| / 7\'7
| \ \   Xilinx Inc.
| / /
| \_\/.\   IBIS Models for VIRTEX-5
[IBIS ver]   3.2
[File name]   dlpc950.ibs
[File Rev]   2.6
[Date]   Tue August 11 14:17:33 2015
[Source]   Derived from spice models, rev0.20, dated 08/17/2007 using
   hspice 2005.03
[Notes]   Xilinx IBIS file for VIRTEX-5 I/O standards.
   All models are preliminary.
   The version of IBISCHK used is ibischk4.
   Ibis models were generated using S2IBIS3.
[Disclaimer] The data in this file is derived from SPICE simulations using
   modeling information extracted from the target process. While
   a great deal of care has been taken to provide information
   that is accurate, this model is considered preliminary as it
   has not been verified by actual silicon measurement. Treat the
   data in this model as preliminary until actual silicon
   verification is performed.
[Copyright]   Copyright 2007, Xilinx Inc., All rights reserved
|   Component VIRTEX-5
[Component]   VIRTEX-5
[Manufacturer]   Xilinx Inc.
[Package]
|FF676
|variable   typ   min   max
R_pkg   311.14m   20.66m   859.35m
L_pkg   3.55nH   0.59nH   9.38nH
C_pkg   2.19pF   0.88pF   4.60pF
[Pin]  signal_name   model_name   R_pin   L_pin   C_pin
G11   dmd_type<0>   LVCMOS25_S_12
G12   dmd_type<1>   LVCMOS25_S_12
H11   dmd_type<2>   LVCMOS25_S_12
H12   dmd_type<3>   LVCMOS25_S_12
AC7   scpclk   LVDCI_33
G10   rst_active   LVCMOS25_S_12
D25   ddcspare0   LVCMOS25_S_12
D26   ddcspare1   LVCMOS25_S_12
B21   dclkin_an   LVDS_25
A7   dclkin_bn   LVDS_25
C21   dclkin_ap   LVDS_25
K20   dclkin_cn   LVDS_25
B7   dclkin_bp   LVDS_25
L5   dclkin_dn   LVDS_25
K21   dclkin_cp   LVDS_25
K5   dclkin_dp   LVDS_25
AD10   reset_strobe   LVDCI_33
A15   din_an<0>   LVDS_25
B14   din_an<1>   LVDS_25
B16   din_an<2>   LVDS_25
C16   din_an<3>   LVDS_25
A17   din_an<4>   LVDS_25
C17   din_an<5>   LVDS_25
A19   din_an<6>   LVDS_25
C18   din_an<7>   LVDS_25
A12   din_bn<0>   LVDS_25
A14   din_ap<0>   LVDS_25
D19   din_an<8>   LVDS_25
B12   din_bn<1>   LVDS_25
C14   din_ap<1>   LVDS_25
B20   din_an<9>   LVDS_25
D10   din_bn<2>   LVDS_25
B15   din_ap<2>   LVDS_25
C12   din_bn<3>   LVDS_25
D16   din_ap<3>   LVDS_25
A10   din_bn<4>   LVDS_25
B17   din_ap<4>   LVDS_25
D9   din_bn<5>   LVDS_25
D18   din_ap<5>   LVDS_25
B10   din_bn<6>   LVDS_25
A18   din_ap<6>   LVDS_25
A8   din_bn<7>   LVDS_25
B19   din_ap<7>   LVDS_25
E20   din_cn<0>   LVDS_25
A13   din_bp<0>   LVDS_25
D6   din_bn<8>   LVDS_25
C19   din_ap<8>   LVDS_25
F20   din_cn<1>   LVDS_25
C13   din_bp<1>   LVDS_25
C7   din_bn<9>   LVDS_25
A20   din_ap<9>   LVDS_25
H19   din_cn<2>   LVDS_25
D11   din_bp<2>   LVDS_25
E23   din_cn<3>   LVDS_25
C11   din_bp<3>   LVDS_25
F23   din_cn<4>   LVDS_25
B11   din_bp<4>   LVDS_25
G22   din_cn<5>   LVDS_25
C9   din_bp<5>   LVDS_25
J20   din_cn<6>   LVDS_25
B9   din_bp<6>   LVDS_25
H22   din_cn<7>   LVDS_25
A9   din_bp<7>   LVDS_25
T3   din_dn<0>   LVDS_25
E21   din_cp<0>   LVDS_25
J23   din_cn<8>   LVDS_25
D5   din_bp<8>   LVDS_25
R5   din_dn<1>   LVDS_25
G20   din_cp<1>   LVDS_25
K22   din_cn<9>   LVDS_25
C6   din_bp<9>   LVDS_25
R7   din_dn<2>   LVDS_25
J19   din_cp<2>   LVDS_25
N3   din_dn<3>   LVDS_25
E22   din_cp<3>   LVDS_25
P4   din_dn<4>   LVDS_25
F22   din_cp<4>   LVDS_25
N6   din_dn<5>   LVDS_25
G21   din_cp<5>   LVDS_25
N4   din_dn<6>   LVDS_25
J21   din_cp<6>   LVDS_25
M7   din_dn<7>   LVDS_25
H21   din_cp<7>   LVDS_25
R3   din_dp<0>   LVDS_25
K7   din_dn<8>   LVDS_25
H23   din_cp<8>   LVDS_25
R6   din_dp<1>   LVDS_25
J4   din_dn<9>   LVDS_25
K23   din_cp<9>   LVDS_25
P6   din_dp<2>   LVDS_25
P3   din_dp<3>   LVDS_25
P5   din_dp<4>   LVDS_25
N7   din_dp<5>   LVDS_25
M4   din_dp<6>   LVDS_25
L7   din_dp<7>   LVDS_25
K6   din_dp<8>   LVDS_25
J5   din_dp<9>   LVDS_25
AD8   reset_irqz   LVCMOS33_S_12
AA10   iic_addr_sel   LVCMOS33_S_12
N1   dclk_an   LVDS_25
Y5   dclk_bn   LVDS_25
M1   dclk_ap   LVDS_25
AA22   dclk_cn   LVDS_25
Y6   dclk_bp   LVDS_25
M26   dclk_dn   LVDS_25
AB22   dclk_cp   LVDS_25
M25   dclk_dp   LVDS_25
H8   speed_sel<0>   LVCMOS25_S_12
H9   speed_sel<1>   LVCMOS25_S_12
G19   comp_data   LVCMOS25_S_12
AA8   iic_sda   LVCMOS33_S_12
E10   clk_r   LVCMOS25_S_12
Y8   iic_scl   LVCMOS33_S_12
F9   arstz   LVCMOS25_S_12
AC8   scpdi   LVCMOS33_S_12
D20   dvalid_an   LVDS_25
C8   dvalid_bn   LVDS_25
D21   dvalid_ap   LVDS_25
L19   dvalid_cn   LVDS_25
D8   dvalid_bp   LVDS_25
L3   dvalid_dn   LVDS_25
L20   dvalid_cp   LVDS_25
L4   dvalid_dp   LVDS_25
F19   ns_flip   LVCMOS25_S_12
A22   din_an<10>   LVDS_25
A24   din_an<11>   LVDS_25
C23   din_an<12>   LVDS_25
C24   din_an<13>   LVDS_25
A25   din_an<14>   LVDS_25
C26   din_an<15>   LVDS_25
B6   din_bn<10>   LVDS_25
B22   din_ap<10>   LVDS_25
D4   din_bn<11>   LVDS_25
A23   din_ap<11>   LVDS_25
B4   din_bn<12>   LVDS_25
B24   din_ap<12>   LVDS_25
C3   din_bn<13>   LVDS_25
D24   din_ap<13>   LVDS_25
A3   din_bn<14>   LVDS_25
B25   din_ap<14>   LVDS_25
B2   din_bn<15>   LVDS_25
B26   din_ap<15>   LVDS_25
M19   din_cn<10>   LVDS_25
B5   din_bp<10>   LVDS_25
M21   din_cn<11>   LVDS_25
D3   din_bp<11>   LVDS_25
N19   din_cn<12>   LVDS_25
C4   din_bp<12>   LVDS_25
N21   din_cn<13>   LVDS_25
C2   din_bp<13>   LVDS_25
P20   din_cn<14>   LVDS_25
A2   din_bp<14>   LVDS_25
N23   din_cn<15>   LVDS_25
B1   din_bp<15>   LVDS_25
H7   din_dn<10>   LVDS_25
M20   din_cp<10>   LVDS_25
G4   din_dn<11>   LVDS_25
M22   din_cp<11>   LVDS_25
G5   din_dn<12>   LVDS_25
P19   din_cp<12>   LVDS_25
G7   din_dn<13>   LVDS_25
N22   din_cp<13>   LVDS_25
F4   din_dn<14>   LVDS_25
P21   din_cp<14>   LVDS_25
E5   din_dn<15>   LVDS_25
P23   din_cp<15>   LVDS_25
J6   din_dp<10>   LVDS_25
H4   din_dp<11>   LVDS_25
H6   din_dp<12>   LVDS_25
G6   din_dp<13>   LVDS_25
F5   din_dp<14>   LVDS_25
E6   din_dp<15>   LVDS_25
AA9   reserved<0>   LVCMOS33_S_12
Y10   reserved<1>   LVCMOS33_S_12
Y11   reserved<2>   LVCMOS33_S_12
AB11   reserved<3>   LVCMOS33_S_12
F18   version<0>   LVCMOS25_S_12
G17   version<1>   LVCMOS25_S_12
H18   version<2>   LVCMOS25_S_12
E1   tstpt_u<10>   LVCMOS25_S_12
E2   tstpt_u<11>   LVCMOS25_S_12
E3   tstpt_u<12>   LVCMOS25_S_12
F3   tstpt_u<13>   LVCMOS25_S_12
E7   tstpt_u<14>   LVCMOS25_S_12
F7   tstpt_u<15>   LVCMOS25_S_12
AD11   dad_spare_scpenz   LVCMOS33_S_12
AC9   scpdo   LVDCI_33
AA17   led0   LVCMOS33_S_12
AB17   led1   LVCMOS33_S_12
E12   blkad<0>   LVCMOS25_S_12
D13   blkad<1>   LVCMOS25_S_12
E13   blkad<2>   LVCMOS25_S_12
F13   blkad<3>   LVCMOS25_S_12
K1   dout_an<10>   LVDS_25
K2   dout_an<11>   LVDS_25
J3   dout_an<12>   LVDS_25
H2   dout_an<13>   LVDS_25
H1   dout_an<14>   LVDS_25
G2   dout_an<15>   LVDS_25
W6   dout_bn<10>   LVDS_25
L2   dout_ap<10>   LVDS_25
V7   dout_bn<11>   LVDS_25
K3   dout_ap<11>   LVDS_25
U4   dout_bn<12>   LVDS_25
H3   dout_ap<12>   LVDS_25
T4   dout_bn<13>   LVDS_25
J1   dout_ap<13>   LVDS_25
U6   dout_bn<14>   LVDS_25
G1   dout_ap<14>   LVDS_25
U7   dout_bn<15>   LVDS_25
F2   dout_ap<15>   LVDS_25
Y20   dout_cn<10>   LVDS_25
W5   dout_bp<10>   LVDS_25
AA24   dout_cn<11>   LVDS_25
V6   dout_bp<11>   LVDS_25
AA19   dout_cn<12>   LVDS_25
V3   dout_bp<12>   LVDS_25
AC24   dout_cn<13>   LVDS_25
T5   dout_bp<13>   LVDS_25
AC19   dout_cn<14>   LVDS_25
U5   dout_bp<14>   LVDS_25
AC22   dout_cn<15>   LVDS_25
T7   dout_bp<15>   LVDS_25
L25   dout_dn<10>   LVDS_25
Y21   dout_cp<10>   LVDS_25
K26   dout_dn<11>   LVDS_25
AA23   dout_cp<11>   LVDS_25
J26   dout_dn<12>   LVDS_25
AA20   dout_cp<12>   LVDS_25
J24   dout_dn<13>   LVDS_25
AB24   dout_cp<13>   LVDS_25
H26   dout_dn<14>   LVDS_25
AD19   dout_cp<14>   LVDS_25
G25   dout_dn<15>   LVDS_25
AC23   dout_cp<15>   LVDS_25
L24   dout_dp<10>   LVDS_25
K25   dout_dp<11>   LVDS_25
J25   dout_dp<12>   LVDS_25
H24   dout_dp<13>   LVDS_25
G26   dout_dp<14>   LVDS_25
G24   dout_dp<15>   LVDS_25
H13   blkmd<0>   LVCMOS25_S_12
H14   blkmd<1>   LVCMOS25_S_12
AB9   dmdscpenz   LVDCI_33
G16   rowad<10>   LVCMOS25_S_12
AB10   dmd_a_reset   LVDCI_33
E26   init_active   LVCMOS25_S_12
AD18   reset_addr<0>   LVDCI_33
AC18   reset_addr<1>   LVDCI_33
AC17   reset_addr<2>   LVDCI_33
AC16   reset_addr<3>   LVDCI_33
E25   ecp2_finished   LVCMOS25_S_12
E8   vsp_en   LVCMOS25_S_12
Y12   tstpt_u<0>   LVCMOS33_S_12
AA12   tstpt_u<1>   LVCMOS33_S_12
Y13   tstpt_u<2>   LVCMOS33_S_12
AA13   tstpt_u<3>   LVCMOS33_S_12
AA14   tstpt_u<4>   LVCMOS33_S_12
AB14   tstpt_u<5>   LVCMOS33_S_12
AA15   tstpt_u<6>   LVCMOS33_S_12
AB15   tstpt_u<7>   LVCMOS33_S_12
C1   tstpt_u<8>   LVCMOS25_S_12
D1   tstpt_u<9>   LVCMOS25_S_12
G9   pwr_float   LVCMOS25_S_12
AD14   reset_oez   LVDCI_33
AE2   dout_an<0>   LVDS_25
AD1   dout_an<1>   LVDS_25
AC1   dout_an<2>   LVDS_25
AB1   dout_an<3>   LVDS_25
Y2   dout_an<4>   LVDS_25
W1   dout_an<5>   LVDS_25
V1   dout_an<6>   LVDS_25
U1   dout_an<7>   LVDS_25
AC13   reset_mode<0>   LVDCI_33
AE5   dout_bn<0>   LVDS_25
AF2   dout_ap<0>   LVDS_25
R2   dout_an<8>   LVDS_25
AD13   reset_mode<1>   LVDCI_33
F25   wdt_enablez   LVCMOS25_S_12
AD3   dout_bn<1>   LVDS_25
AE1   dout_ap<1>   LVDS_25
N2   dout_an<9>   LVDS_25
AD5   dout_bn<2>   LVDS_25
AC2   dout_ap<2>   LVDS_25
AC3   dout_bn<3>   LVDS_25
AB2   dout_ap<3>   LVDS_25
AB5   dout_bn<4>   LVDS_25
AA2   dout_ap<4>   LVDS_25
AB7   dout_bn<5>   LVDS_25
Y1   dout_ap<5>   LVDS_25
AA5   dout_bn<6>   LVDS_25
V2   dout_ap<6>   LVDS_25
AA7   dout_bn<7>   LVDS_25
U2   dout_ap<7>   LVDS_25
T22   dout_cn<0>   LVDS_25
AE6   dout_bp<0>   LVDS_25
Y3   dout_bn<8>   LVDS_25
T2   dout_ap<8>   LVDS_25
R20   dout_cn<1>   LVDS_25
AD4   dout_bp<1>   LVDS_25
W4   dout_bn<9>   LVDS_25
M2   dout_ap<9>   LVDS_25
T19   dout_cn<2>   LVDS_25
AD6   dout_bp<2>   LVDS_25
U21   dout_cn<3>   LVDS_25
AC4   dout_bp<3>   LVDS_25
U20   dout_cn<4>   LVDS_25
AB6   dout_bp<4>   LVDS_25
V23   dout_cn<5>   LVDS_25
AC6   dout_bp<5>   LVDS_25
V22   dout_cn<6>   LVDS_25
AA4   dout_bp<6>   LVDS_25
W19   dout_cn<7>   LVDS_25
Y7   dout_bp<7>   LVDS_25
AB26   dout_dn<0>   LVDS_25
T23   dout_cp<0>   LVDS_25
W23   dout_cn<8>   LVDS_25
W3   dout_bp<8>   LVDS_25
AA25   dout_dn<1>   LVDS_25
R21   dout_cp<1>   LVDS_25
Y22   dout_cn<9>   LVDS_25
V4   dout_bp<9>   LVDS_25
Y26   dout_dn<2>   LVDS_25
T20   dout_cp<2>   LVDS_25
W26   dout_dn<3>   LVDS_25
U22   dout_cp<3>   LVDS_25
U26   dout_dn<4>   LVDS_25
U19   dout_cp<4>   LVDS_25
U25   dout_dn<5>   LVDS_25
V24   dout_cp<5>   LVDS_25
T25   dout_dn<6>   LVDS_25
V21   dout_cp<6>   LVDS_25
R26   dout_dn<7>   LVDS_25
V19   dout_cp<7>   LVDS_25
AC26   dout_dp<0>   LVDS_25
P24   dout_dn<8>   LVDS_25
W24   dout_cp<8>   LVDS_25
AB25   dout_dp<1>   LVDS_25
N24   dout_dn<9>   LVDS_25
Y23   dout_cp<9>   LVDS_25
Y25   dout_dp<2>   LVDS_25
W25   dout_dp<3>   LVDS_25
V26   dout_dp<4>   LVDS_25
U24   dout_dp<5>   LVDS_25
T24   dout_dp<6>   LVDS_25
R25   dout_dp<7>   LVDS_25
P25   dout_dp<8>   LVDS_25
M24   dout_dp<9>   LVDS_25
E18   rst2blkz   LVCMOS25_S_12
R1   sctrl_an   LVDS_25
AA3   sctrl_bn   LVDS_25
P1   sctrl_ap   LVDS_25
W20   sctrl_cn   LVDS_25
AB4   sctrl_bp   LVDS_25
N26   sctrl_dn   LVDS_25
W21   sctrl_cp   LVDS_25
P26   sctrl_dp   LVDS_25
D14   rowad<0>   LVCMOS25_S_12
D15   rowad<1>   LVCMOS25_S_12
E15   rowad<2>   LVCMOS25_S_12
F14   rowad<3>   LVCMOS25_S_12
G14   rowad<4>   LVCMOS25_S_12
E16   rowad<5>   LVCMOS25_S_12
F15   rowad<6>   LVCMOS25_S_12
G15   rowad<7>   LVCMOS25_S_12
E17   rowad<8>   LVCMOS25_S_12
F17   rowad<9>   LVCMOS25_S_12
H17   rowmd<0>   LVCMOS25_S_12
H16   rowmd<1>   LVCMOS25_S_12
AD15   reset_sel<0>   LVDCI_33
AC14   reset_sel<1>   LVDCI_33
AC12   dad_scpenz   LVCMOS33_S_12
F8   reserved_clk   LVCMOS25_S_12
N14   VP_0   NC
P13   VN_0   NC
AA18   A25   LVCMOS25_F_12
Y18   A24   LVCMOS25_F_12
AB16   CSO_B   LVCMOS25_F_12
F12   IO_L2N_GC_VRP_3   NC
E11   IO_L4N_GC_VREF_3   NC
F10   IO_L6N_GC_3   NC
AB12   IO_L7P_GC_VRN_4   NC
AC11   IO_L7N_GC_VRP_4   NC
L23   IO_L12P_VRN_11   NC
L22   IO_L12N_VRP_11   NC
R22   SM10P   NC
R23   SM10N   NC
M5   IO_L12P_VRN_12   NC
M6   IO_L12N_VRP_12   NC
F24   SM8P   NC
D23   IO_L12P_VRN_15   NC
C22   IO_L12N_VRP_15   NC
A4   IO_L12P_VRN_16   NC
A5   IO_L12N_VRP_16   NC
AC21   IO_L11P_CC_17   NC
AB21   IO_L11N_CC_17   NC
AB20   IO_L18P_17   NC
AB19   IO_L18N_17   NC
AF3   IO_L16P_18   NC
AE3   IO_L16N_18   NC
AF5   IO_L18P_18   NC
AF4   IO_L18N_18   NC
R14   DXP_0   NC
R13   DXN_0   NC
M14   AVDD_0   NC
M13   AVSS_0   NC
P14   VREFP_0   NC
N13   VREFN_0   NC
K18   VBATT_0   NC
J18   PROGRAM_B_0   NC
L18   HSWAPEN_0   NC
K11   D_IN_0   NC
K10   DONE_0   NC
J10   CCLK_0   NC
J11   INIT_B_0   NC
N18   CS_B_0   NC
P18   RDWR_B_0   NC
R18   RSVD_0   NC
T18   RSVD_0   NC
U11   TCK_0   NC
W18   M0_0   NC
V18   M2_0   NC
Y17   M1_0   NC
V12   TMS_0   NC
V11   TDI_0   NC
W11   D_OUT_BUSY_0   NC
W10   TDO_0   NC
A1   GND   GND
F1   GND   GND
L1   GND   GND
T1   GND   GND
AA1   GND   GND
AF1   GND   GND
D2   GND   GND
P2   GND   GND
AD2   GND   GND
B3   GND   GND
G3   GND   GND
M3   GND   GND
U3   GND   GND
K4   GND   GND
Y4   GND   GND
AE4   GND   GND
C5   GND   GND
N5   GND   GND
AC5   GND   GND
A6   GND   GND
F6   GND   GND
T6   GND   GND
AF6   GND   GND
J7   GND   GND
P7   GND   GND
W7   GND   GND
B8   GND   GND
K8   GND   GND
M8   GND   GND
P8   GND   GND
T8   GND   GND
V8   GND   GND
AB8   GND   GND
E9   GND   GND
J9   GND   GND
L9   GND   GND
N9   GND   GND
R9   GND   GND
U9   GND   GND
W9   GND   GND
AE9   GND   GND
H10   GND   GND
M10   GND   GND
P10   GND   GND
T10   GND   GND
V10   GND   GND
A11   GND   GND
L11   GND   GND
N11   GND   GND
R11   GND   GND
AA11   GND   GND
AF11   GND   GND
D12   GND   GND
K12   GND   GND
M12   GND   GND
P12   GND   GND
T12   GND   GND
AD12   GND   GND
B13   GND   GND
G13   GND   GND
J13   GND   GND
L13   GND   GND
U13   GND   GND
W13   GND   GND
K14   GND   GND
T14   GND   GND
V14   GND   GND
Y14   GND   GND
AE14   GND   GND
C15   GND   GND
J15   GND   GND
L15   GND   GND
N15   GND   GND
R15   GND   GND
U15   GND   GND
W15   GND   GND
AC15   GND   GND
A16   GND   GND
F16   GND   GND
K16   GND   GND
M16   GND   GND
P16   GND   GND
T16   GND   GND
V16   GND   GND
Y16   GND   GND
AF16   GND   GND
J17   GND   GND
L17   GND   GND
N17   GND   GND
R17   GND   GND
U17   GND   GND
W17   GND   GND
B18   GND   GND
G18   GND   GND
M18   GND   GND
U18   GND   GND
AB18   GND   GND
E19   GND   GND
K19   GND   GND
R19   GND   GND
Y19   GND   GND
AE19   GND   GND
H20   GND   GND
V20   GND   GND
A21   GND   GND
L21   GND   GND
AA21   GND   GND
AF21   GND   GND
D22   GND   GND
P22   GND   GND
AD22   GND   GND
G23   GND   GND
U23   GND   GND
K24   GND   GND
Y24   GND   GND
C25   GND   GND
N25   GND   GND
AC25   GND   GND
A26   GND   GND
F26   GND   GND
L26   GND   GND
T26   GND   GND
AA26   GND   GND
AF26   GND   GND
J8   VCCAUX   POWER
L8   VCCAUX   POWER
N8   VCCAUX   POWER
R8   VCCAUX   POWER
U8   VCCAUX   POWER
W8   VCCAUX   POWER
W16   VCCAUX   POWER
K17   VCCAUX   POWER
M17   VCCAUX   POWER
P17   VCCAUX   POWER
T17   VCCAUX   POWER
V17   VCCAUX   POWER
K9   VCCINT   POWER
M9   VCCINT   POWER
P9   VCCINT   POWER
T9   VCCINT   POWER
V9   VCCINT   POWER
L10   VCCINT   POWER
N10   VCCINT   POWER
R10   VCCINT   POWER
U10   VCCINT   POWER
M11   VCCINT   POWER
P11   VCCINT   POWER
T11   VCCINT   POWER
J12   VCCINT   POWER
L12   VCCINT   POWER
N12   VCCINT   POWER
R12   VCCINT   POWER
U12   VCCINT   POWER
K13   VCCINT   POWER
T13   VCCINT   POWER
V13   VCCINT   POWER
J14   VCCINT   POWER
L14   VCCINT   POWER
U14   VCCINT   POWER
W14   VCCINT   POWER
H15   VCCINT   POWER
K15   VCCINT   POWER
M15   VCCINT   POWER
P15   VCCINT   POWER
T15   VCCINT   POWER
V15   VCCINT   POWER
Y15   VCCINT   POWER
J16   VCCINT   POWER
L16   VCCINT   POWER
N16   VCCINT   POWER
U16   VCCINT   POWER
R16   VCCINT   POWER
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[Package Model]   ff676_xc5vlx30
[Diff Pin]   inv_pin   vdiff   tdelay_typ   tdelay_min   tdelay_max
M1   N1   100mV   0   0   0
| dclk_ap   LVDS_25   LVDS_25
Y6   Y5   100mV   0   0   0
| dclk_bp   LVDS_25   LVDS_25
AB22   AA22   100mV   0   0   0
| dclk_cp   LVDS_25   LVDS_25
M25   M26   100mV   0   0   0
| dclk_dp   LVDS_25   LVDS_25
L2   K1   100mV   0   0   0
| dout_ap<10>   LVDS_25   LVDS_25
K3   K2   100mV   0   0   0
| dout_ap<11>   LVDS_25   LVDS_25
H3   J3   100mV   0   0   0
| dout_ap<12>   LVDS_25   LVDS_25
J1   H2   100mV   0   0   0
| dout_ap<13>   LVDS_25   LVDS_25
G1   H1   100mV   0   0   0
| dout_ap<14>   LVDS_25   LVDS_25
F2   G2   100mV   0   0   0
| dout_ap<15>   LVDS_25   LVDS_25
W5   W6   100mV   0   0   0
| dout_bp<10>   LVDS_25   LVDS_25
V6   V7   100mV   0   0   0
| dout_bp<11>   LVDS_25   LVDS_25
V3   U4   100mV   0   0   0
| dout_bp<12>   LVDS_25   LVDS_25
T5   T4   100mV   0   0   0
| dout_bp<13>   LVDS_25   LVDS_25
U5   U6   100mV   0   0   0
| dout_bp<14>   LVDS_25   LVDS_25
T7   U7   100mV   0   0   0
| dout_bp<15>   LVDS_25   LVDS_25
Y21   Y20   100mV   0   0   0
| dout_cp<10>   LVDS_25   LVDS_25
AA23   AA24   100mV   0   0   0
| dout_cp<11>   LVDS_25   LVDS_25
AA20   AA19   100mV   0   0   0
| dout_cp<12>   LVDS_25   LVDS_25
AB24   AC24   100mV   0   0   0
| dout_cp<13>   LVDS_25   LVDS_25
AD19   AC19   100mV   0   0   0
| dout_cp<14>   LVDS_25   LVDS_25
AC23   AC22   100mV   0   0   0
| dout_cp<15>   LVDS_25   LVDS_25
L24   L25   100mV   0   0   0
| dout_dp<10>   LVDS_25   LVDS_25
K25   K26   100mV   0   0   0
| dout_dp<11>   LVDS_25   LVDS_25
J25   J26   100mV   0   0   0
| dout_dp<12>   LVDS_25   LVDS_25
H24   J24   100mV   0   0   0
| dout_dp<13>   LVDS_25   LVDS_25
G26   H26   100mV   0   0   0
| dout_dp<14>   LVDS_25   LVDS_25
G24   G25   100mV   0   0   0
| dout_dp<15>   LVDS_25   LVDS_25
AF2   AE2   100mV   0   0   0
| dout_ap<0>   LVDS_25   LVDS_25
AE1   AD1   100mV   0   0   0
| dout_ap<1>   LVDS_25   LVDS_25
AC2   AC1   100mV   0   0   0
| dout_ap<2>   LVDS_25   LVDS_25
AB2   AB1   100mV   0   0   0
| dout_ap<3>   LVDS_25   LVDS_25
AA2   Y2   100mV   0   0   0
| dout_ap<4>   LVDS_25   LVDS_25
Y1   W1   100mV   0   0   0
| dout_ap<5>   LVDS_25   LVDS_25
V2   V1   100mV   0   0   0
| dout_ap<6>   LVDS_25   LVDS_25
U2   U1   100mV   0   0   0
| dout_ap<7>   LVDS_25   LVDS_25
AE6   AE5   100mV   0   0   0
| dout_bp<0>   LVDS_25   LVDS_25
T2   R2   100mV   0   0   0
| dout_ap<8>   LVDS_25   LVDS_25
AD4   AD3   100mV   0   0   0
| dout_bp<1>   LVDS_25   LVDS_25
M2   N2   100mV   0   0   0
| dout_ap<9>   LVDS_25   LVDS_25
AD6   AD5   100mV   0   0   0
| dout_bp<2>   LVDS_25   LVDS_25
AC4   AC3   100mV   0   0   0
| dout_bp<3>   LVDS_25   LVDS_25
AB6   AB5   100mV   0   0   0
| dout_bp<4>   LVDS_25   LVDS_25
AC6   AB7   100mV   0   0   0
| dout_bp<5>   LVDS_25   LVDS_25
AA4   AA5   100mV   0   0   0
| dout_bp<6>   LVDS_25   LVDS_25
Y7   AA7   100mV   0   0   0
| dout_bp<7>   LVDS_25   LVDS_25
T23   T22   100mV   0   0   0
| dout_cp<0>   LVDS_25   LVDS_25
W3   Y3   100mV   0   0   0
| dout_bp<8>   LVDS_25   LVDS_25
R21   R20   100mV   0   0   0
| dout_cp<1>   LVDS_25   LVDS_25
V4   W4   100mV   0   0   0
| dout_bp<9>   LVDS_25   LVDS_25
T20   T19   100mV   0   0   0
| dout_cp<2>   LVDS_25   LVDS_25
U22   U21   100mV   0   0   0
| dout_cp<3>   LVDS_25   LVDS_25
U19   U20   100mV   0   0   0
| dout_cp<4>   LVDS_25   LVDS_25
V24   V23   100mV   0   0   0
| dout_cp<5>   LVDS_25   LVDS_25
V21   V22   100mV   0   0   0
| dout_cp<6>   LVDS_25   LVDS_25
V19   W19   100mV   0   0   0
| dout_cp<7>   LVDS_25   LVDS_25
AC26   AB26   100mV   0   0   0
| dout_dp<0>   LVDS_25   LVDS_25
W24   W23   100mV   0   0   0
| dout_cp<8>   LVDS_25   LVDS_25
AB25   AA25   100mV   0   0   0
| dout_dp<1>   LVDS_25   LVDS_25
Y23   Y22   100mV   0   0   0
| dout_cp<9>   LVDS_25   LVDS_25
Y25   Y26   100mV   0   0   0
| dout_dp<2>   LVDS_25   LVDS_25
W25   W26   100mV   0   0   0
| dout_dp<3>   LVDS_25   LVDS_25
V26   U26   100mV   0   0   0
| dout_dp<4>   LVDS_25   LVDS_25
U24   U25   100mV   0   0   0
| dout_dp<5>   LVDS_25   LVDS_25
T24   T25   100mV   0   0   0
| dout_dp<6>   LVDS_25   LVDS_25
R25   R26   100mV   0   0   0
| dout_dp<7>   LVDS_25   LVDS_25
P25   P24   100mV   0   0   0
| dout_dp<8>   LVDS_25   LVDS_25
M24   N24   100mV   0   0   0
| dout_dp<9>   LVDS_25   LVDS_25
P1   R1   100mV   0   0   0
| sctrl_ap   LVDS_25   LVDS_25
AB4   AA3   100mV   0   0   0
| sctrl_bp   LVDS_25   LVDS_25
W21   W20   100mV   0   0   0
| sctrl_cp   LVDS_25   LVDS_25
P26   N26   100mV   0   0   0
| sctrl_dp   LVDS_25   LVDS_25
C21   B21   100mV   0   0   0
| dclkin_ap   LVDS_25_DT   LVDS_25
B7   A7   100mV   0   0   0
| dclkin_bp   LVDS_25_DT   LVDS_25
K21   K20   100mV   0   0   0
| dclkin_cp   LVDS_25_DT   LVDS_25
K5   L5   100mV   0   0   0
| dclkin_dp   LVDS_25_DT   LVDS_25
A14   A15   100mV   0   0   0
| din_ap<0>   LVDS_25_DT   LVDS_25
C14   B14   100mV   0   0   0
| din_ap<1>   LVDS_25_DT   LVDS_25
B15   B16   100mV   0   0   0
| din_ap<2>   LVDS_25_DT   LVDS_25
D16   C16   100mV   0   0   0
| din_ap<3>   LVDS_25_DT   LVDS_25
B17   A17   100mV   0   0   0
| din_ap<4>   LVDS_25_DT   LVDS_25
D18   C17   100mV   0   0   0
| din_ap<5>   LVDS_25_DT   LVDS_25
A18   A19   100mV   0   0   0
| din_ap<6>   LVDS_25_DT   LVDS_25
B19   C18   100mV   0   0   0
| din_ap<7>   LVDS_25_DT   LVDS_25
A13   A12   100mV   0   0   0
| din_bp<0>   LVDS_25_DT   LVDS_25
C19   D19   100mV   0   0   0
| din_ap<8>   LVDS_25_DT   LVDS_25
C13   B12   100mV   0   0   0
| din_bp<1>   LVDS_25_DT   LVDS_25
A20   B20   100mV   0   0   0
| din_ap<9>   LVDS_25_DT   LVDS_25
D11   D10   100mV   0   0   0
| din_bp<2>   LVDS_25_DT   LVDS_25
C11   C12   100mV   0   0   0
| din_bp<3>   LVDS_25_DT   LVDS_25
B11   A10   100mV   0   0   0
| din_bp<4>   LVDS_25_DT   LVDS_25
C9   D9   100mV   0   0   0
| din_bp<5>   LVDS_25_DT   LVDS_25
B9   B10   100mV   0   0   0
| din_bp<6>   LVDS_25_DT   LVDS_25
A9   A8   100mV   0   0   0
| din_bp<7>   LVDS_25_DT   LVDS_25
E21   E20   100mV   0   0   0
| din_cp<0>   LVDS_25_DT   LVDS_25
D5   D6   100mV   0   0   0
| din_bp<8>   LVDS_25_DT   LVDS_25
G20   F20   100mV   0   0   0
| din_cp<1>   LVDS_25_DT   LVDS_25
C6   C7   100mV   0   0   0
| din_bp<9>   LVDS_25_DT   LVDS_25
J19   H19   100mV   0   0   0
| din_cp<2>   LVDS_25_DT   LVDS_25
E22   E23   100mV   0   0   0
| din_cp<3>   LVDS_25_DT   LVDS_25
F22   F23   100mV   0   0   0
| din_cp<4>   LVDS_25_DT   LVDS_25
G21   G22   100mV   0   0   0
| din_cp<5>   LVDS_25_DT   LVDS_25
J21   J20   100mV   0   0   0
| din_cp<6>   LVDS_25_DT   LVDS_25
H21   H22   100mV   0   0   0
| din_cp<7>   LVDS_25_DT   LVDS_25
R3   T3   100mV   0   0   0
| din_dp<0>   LVDS_25_DT   LVDS_25
H23   J23   100mV   0   0   0
| din_cp<8>   LVDS_25_DT   LVDS_25
R6   R5   100mV   0   0   0
| din_dp<1>   LVDS_25_DT   LVDS_25
K23   K22   100mV   0   0   0
| din_cp<9>   LVDS_25_DT   LVDS_25
P6   R7   100mV   0   0   0
| din_dp<2>   LVDS_25_DT   LVDS_25
P3   N3   100mV   0   0   0
| din_dp<3>   LVDS_25_DT   LVDS_25
P5   P4   100mV   0   0   0
| din_dp<4>   LVDS_25_DT   LVDS_25
N7   N6   100mV   0   0   0
| din_dp<5>   LVDS_25_DT   LVDS_25
M4   N4   100mV   0   0   0
| din_dp<6>   LVDS_25_DT   LVDS_25
L7   M7   100mV   0   0   0
| din_dp<7>   LVDS_25_DT   LVDS_25
K6   K7   100mV   0   0   0
| din_dp<8>   LVDS_25_DT   LVDS_25
J5   J4   100mV   0   0   0
| din_dp<9>   LVDS_25_DT   LVDS_25
D21   D20   100mV   0   0   0
| dvalid_ap   LVDS_25_DT   LVDS_25
D8   C8   100mV   0   0   0
| dvalid_bp   LVDS_25_DT   LVDS_25
L20   L19   100mV   0   0   0
| dvalid_cp   LVDS_25_DT   LVDS_25
L4   L3   100mV   0   0   0
| dvalid_dp   LVDS_25_DT   LVDS_25
B22   A22   100mV   0   0   0
| din_ap<10>   LVDS_25_DT   LVDS_25
A23   A24   100mV   0   0   0
| din_ap<11>   LVDS_25_DT   LVDS_25
B24   C23   100mV   0   0   0
| din_ap<12>   LVDS_25_DT   LVDS_25
D24   C24   100mV   0   0   0
| din_ap<13>   LVDS_25_DT   LVDS_25
B25   A25   100mV   0   0   0
| din_ap<14>   LVDS_25_DT   LVDS_25
B26   C26   100mV   0   0   0
| din_ap<15>   LVDS_25_DT   LVDS_25
B5   B6   100mV   0   0   0
| din_bp<10>   LVDS_25_DT   LVDS_25
D3   D4   100mV   0   0   0
| din_bp<11>   LVDS_25_DT   LVDS_25
C4   B4   100mV   0   0   0
| din_bp<12>   LVDS_25_DT   LVDS_25
C2   C3   100mV   0   0   0
| din_bp<13>   LVDS_25_DT   LVDS_25
A2   A3   100mV   0   0   0
| din_bp<14>   LVDS_25_DT   LVDS_25
B1   B2   100mV   0   0   0
| din_bp<15>   LVDS_25_DT   LVDS_25
M20   M19   100mV   0   0   0
| din_cp<10>   LVDS_25_DT   LVDS_25
M22   M21   100mV   0   0   0
| din_cp<11>   LVDS_25_DT   LVDS_25
P19   N19   100mV   0   0   0
| din_cp<12>   LVDS_25_DT   LVDS_25
N22   N21   100mV   0   0   0
| din_cp<13>   LVDS_25_DT   LVDS_25
P21   P20   100mV   0   0   0
| din_cp<14>   LVDS_25_DT   LVDS_25
P23   N23   100mV   0   0   0
| din_cp<15>   LVDS_25_DT   LVDS_25
J6   H7   100mV   0   0   0
| din_dp<10>   LVDS_25_DT   LVDS_25
H4   G4   100mV   0   0   0
| din_dp<11>   LVDS_25_DT   LVDS_25
H6   G5   100mV   0   0   0
| din_dp<12>   LVDS_25_DT   LVDS_25
G6   G7   100mV   0   0   0
| din_dp<13>   LVDS_25_DT   LVDS_25
F5   F4   100mV   0   0   0
| din_dp<14>   LVDS_25_DT   LVDS_25
E6   E5   100mV   0   0   0
| din_dp<15>   LVDS_25_DT   LVDS_25
[Series Pin Mapping] pin_2   model_name   function_table_group
C21   B21   rterm_100
B7   A7   rterm_100
K21   K20   rterm_100
K5   L5   rterm_100
A14   A15   rterm_100
C14   B14   rterm_100
B15   B16   rterm_100
D16   C16   rterm_100
B17   A17   rterm_100
D18   C17   rterm_100
A18   A19   rterm_100
B19   C18   rterm_100
A13   A12   rterm_100
C19   D19   rterm_100
C13   B12   rterm_100
A20   B20   rterm_100
D11   D10   rterm_100
C11   C12   rterm_100
B11   A10   rterm_100
C9   D9   rterm_100
B9   B10   rterm_100
A9   A8   rterm_100
E21   E20   rterm_100
D5   D6   rterm_100
G20   F20   rterm_100
C6   C7   rterm_100
J19   H19   rterm_100
E22   E23   rterm_100
F22   F23   rterm_100
G21   G22   rterm_100
J21   J20   rterm_100
H21   H22   rterm_100
R3   T3   rterm_100
H23   J23   rterm_100
R6   R5   rterm_100
K23   K22   rterm_100
P6   R7   rterm_100
P3   N3   rterm_100
P5   P4   rterm_100
N7   N6   rterm_100
M4   N4   rterm_100
L7   M7   rterm_100
K6   K7   rterm_100
J5   J4   rterm_100
D21   D20   rterm_100
D8   C8   rterm_100
L20   L19   rterm_100
L4   L3   rterm_100
B22   A22   rterm_100
A23   A24   rterm_100
B24   C23   rterm_100
D24   C24   rterm_100
B25   A25   rterm_100
B26   C26   rterm_100
B5   B6   rterm_100
D3   D4   rterm_100
C4   B4   rterm_100
C2   C3   rterm_100
A2   A3   rterm_100
B1   B2   rterm_100
M20   M19   rterm_100
M22   M21   rterm_100
P19   N19   rterm_100
N22   N21   rterm_100
P21   P20   rterm_100
P23   N23   rterm_100
J6   H7   rterm_100
H4   G4   rterm_100
H6   G5   rterm_100
G6   G7   rterm_100
F5   F4   rterm_100
E6   E5   rterm_100
[Define Package Model]   ff676_xc5vlx30
[Manufacturer]   Xilinx Inc.
[OEM]   Xilinx_K1
[Description]   676 ball organic flipchip
[Number Of Pins]   444
[Pin Numbers]
P20   | 1   P20   D1.245   IO_L19N_SM9N_11
AC17   | 2   AC17  D1.164   IO_L2P_GC_D11_4
F18   | 3   F18   D1.145   IO_L9P_GC_3
B12   | 4   B12   D1.534   IO_L2N_16
T19   | 5   T19   D1.603   IO_L2N_17
H1   | 6   H1   D1.399   IO_L2N_14
B16   | 7   B16   D1.468   IO_L2N_15
G7   | 8   G7   D1.264   IO_L2N_12
E23   | 9   E23   D1.198   IO_L2N_11
K25   | 10   K25   D1.342   IO_L7P_SM2P_13
U6   | 11   U6   D1.671   IO_L3N_18
U21   | 12   U21   D1.605   IO_L3N_17
A12   | 13   A12   D1.536   IO_L3N_16
C16   | 14   C16   D1.470   IO_L3N_15
G2   | 15   G2   D1.401   IO_L3N_14
F4   | 16   F4   D1.266   IO_L3N_12
F23   | 17   F23   D1.200   IO_L3N_11
F10   | 18   F10   D1.140   IO_L6N_GC_3
J18   | 19   J18   D1.26   PROGRAM_B_0
E8   | 20   E8   D1.144   IO_L8N_GC_3
AC4   | 21   AC4   D1.702   IO_L12P_VRN_18
R25   | 22   R25   D1.365   IO_L12P_VRN_13
M5   | 23   M5   D1.297   IO_L12P_VRN_12
L23   | 24   L23   D1.230   IO_L12P_VRN_11
V21   | 25   V21   D1.635   IO_L12P_VRN_17
A4   | 26   A4   D1.567   IO_L12P_VRN_16
D23   | 27   D23   D1.500   IO_L12P_VRN_15
U2   | 28   U2   D1.432   IO_L12P_VRN_14
K22   | 29   K22   D1.227   IO_L10N_CC_SM15N_11
U7   | 30   U7   D1.669   IO_L2N_18
W12   | 31   W12   D1.35   VCCO_0
C10   | 32   C10   C3.1   VCCO_1
AA16   | 33   AA16  C15.2   VCCO_2
D17   | 34   D17   C4.1   VCCO_3
AB13   | 35   AB13  C16.2   VCCO_4
W11   | 36   W11   D1.59   D_OUT_BUSY_0
M21   | 37   M21   D1.233   IO_L13N_11
T25   | 38   T25   D1.368   IO_L13N_13
N6   | 39   N6   D1.300   IO_L13N_12
A22   | 40   A22   D1.503   IO_L13N_15
V1   | 41   V1   D1.435   IO_L13N_14
W20   | 42   W20   D1.638   IO_L13N_17
B6   | 43   B6   D1.570   IO_L13N_16
L25   | 44   L25   D1.341   IO_L6N_SM3N_13
F19   | 45   F19   D1.142   IO_L7N_GC_3
Y18   | 46   Y18   D1.97   IO_L1N_CC_A24_2
W4   | 47   W4   D1.673   IO_L4N_VREF_18
W24   | 48   W24   D1.606   IO_L4P_17
J26   | 49   J26   D1.337   IO_L4N_VREF_13
H7   | 50   H7   D1.268   IO_L4N_VREF_12
G22   | 51   G22   D1.202   IO_L4N_VREF_11
W23   | 52   W23   D1.607   IO_L4N_VREF_17
D9   | 53   D9   D1.538   IO_L4N_VREF_16
C17   | 54   C17   D1.472   IO_L4N_VREF_15
K2   | 55   K2   D1.403   IO_L4N_VREF_14
H23   | 56   H23   D1.207   IO_L7P_11
J25   | 57   J25   D1.336   IO_L4P_13
U11   | 58   U11   D1.51   TCK_0
J10   | 59   J10   D1.30   CCLK_0
N14   | 60   N14   D1.16   VP_0
AA19   | 61   AA19  D1.650   IO_L19N_17
B2   | 62   B2   D1.582   IO_L19N_16
D25   | 63   D25   D1.515   IO_L19N_15
AE2   | 64   AE2   D1.447   IO_L19N_14
AB26   | 65   AB26  D1.380   IO_L19N_13
R7   | 66   R7   D1.312   IO_L19N_12
G19   | 67   G19   D1.77   IO_L8P_CC_A3_D19_1
AE5   | 68   AE5   D1.717   IO_L19N_18
R4   | 69   R4   C20.1   VCCO_14
G24   | 70   G24   D1.334   IO_L3P_SM5P_13
K11   | 71   K11   D1.28   D_IN_0
B19   | 72   B19   D1.477   IO_L7P_15
AA7   | 73   AA7   D1.699   IO_L10N_CC_18
AC18   | 74   AC18  D1.161   IO_L0N_GC_D14_4
P13   | 75   P13   D1.17   VN_0
AA8   | 76   AA8   D1.99   IO_L2N_A22_2
L5   | 77   L5   D1.294   IO_L10N_CC_12
N26   | 78   N26   D1.362   IO_L10N_CC_13
D6   | 79   D6   D1.564   IO_L10N_CC_16
AA22   | 80   AA22  D1.632   IO_L10N_CC_17
R1   | 81   R1   D1.429   IO_L10N_CC_14
D20   | 82   D20   D1.497   IO_L10N_CC_15
AC14   | 83   AC14  D1.173   IO_L6N_GC_4
F5   | 84   F5   D1.265   IO_L3P_12
D16   | 85   D16   D1.469   IO_L3P_15
P23   | 86   P23   D1.238   IO_L16P_SM12P_11
J5   | 87   J5   D1.273   IO_L7P_12
R18   | 88   R18   D1.38   VFS_0
C24   | 89   C24   D1.509   IO_L16N_15
F12   | 90   F12   D1.132   IO_L2N_GC_VRP_3
H5   | 91   H5   C22.1   VCCO_12
M23   | 92   M23   C9.2   VCCO_13
F21   | 93   F21   C8.2   VCCO_11
D7   | 94   D7   C1.1   VCCO_16
T21   | 95   T21   C11.2   VCCO_17
H14   | 96   H14   D1.63   IO_L1P_A17_1
B23   | 97   B23   C6.1   VCCO_15
AA6   | 98   AA6   C18.2   VCCO_18
K23   | 99   K23   D1.226   IO_L10P_CC_SM15P_11
AD18   | 100   AD18  D1.160   IO_L0P_GC_D15_4
AD4   | 101   AD4   D1.704   IO_L13P_18
K26   | 102   K26   D1.343   IO_L7N_SM2N_13
U24   | 103   U24   D1.371   IO_L15P_13
M4   | 104   M4   D1.303   IO_L15P_12
B24   | 105   B24   D1.506   IO_L15P_15
AA2   | 106   AA2   D1.438   IO_L15P_14
V19   | 107   V19   D1.641   IO_L15P_17
C4   | 108   C4   D1.573   IO_L15P_16
AC6   | 109   AC6   D1.708   IO_L15P_18
C7   | 110   C7   D1.566   IO_L11N_CC_16
V18   | 111   V18   D1.55   M2_0
G25   | 112   G25   D1.335   IO_L3N_SM5N_13
G15   | 113   G15   D1.66   IO_L2N_A14_D30_1
J20   | 114   J20   D1.210   IO_L8N_CC_11
K7   | 115   K7   D1.276   IO_L8N_CC_12
N1   | 116   N1   D1.411   IO_L8N_CC_14
B20   | 117   B20   D1.480   IO_L8N_CC_15
C8   | 118   C8   D1.546   IO_L8N_CC_16
AB9   | 119   AB9   D1.163   IO_L1N_GC_D12_4
Y5   | 120   Y5   D1.681   IO_L8N_CC_18
AB12   | 121   AB12  D1.174   IO_L7P_GC_VRN_4
AC12   | 122   AC12  D1.177   IO_L8N_CC_GC_4
AF5   | 123   AF5   D1.714   IO_L18P_18
R6   | 124   R6   D1.309   IO_L18P_12
AB25   | 125   AB25  D1.377   IO_L18P_13
AE1   | 126   AE1   D1.444   IO_L18P_14
B26   | 127   B26   D1.512   IO_L18P_15
D1   | 128   D1   D1.579   IO_L18P_16
AB20   | 129   AB20  D1.647   IO_L18P_17
L19   | 130   L19   D1.229   IO_L11N_CC_SM14N_11
H8   | 131   H8   D1.80   IO_L9N_CC_A0_D16_1
AC9   | 132   AC9   D1.167   IO_L3N_GC_D8_4
K10   | 133   K10   D1.29   DONE_0
G26   | 134   G26   D1.332   IO_L2P_SM6P_13
J8   | 135   J8   C10.2   VCCAUX
U25   | 136   U25   D1.372   IO_L15N_13
AA14   | 137   AA14  D1.113   IO_L9N_D0_FS0_2
Y17   | 138   Y17   D1.56   M1_0
W19   | 139   W19   D1.642   IO_L15N_17
B4   | 140   B4   D1.574   IO_L15N_16
C23   | 141   C23   D1.507   IO_L15N_15
Y2   | 142   Y2   D1.439   IO_L15N_14
AB7   | 143   AB7   D1.709   IO_L15N_18
AB6   | 144   AB6   D1.706   IO_L14P_18
Y1   | 145   Y1   D1.436   IO_L14P_14
A23   | 146   A23   D1.504   IO_L14P_15
D3   | 147   D3   D1.571   IO_L14P_16
U19   | 148   U19   D1.639   IO_L14P_17
P19   | 149   P19   D1.234   IO_L14P_11
P3   | 150   P3   D1.301   IO_L14P_12
V26   | 151   V26   D1.369   IO_L14P_13
AD19   | 152   AD19  D1.645   IO_L17P_17
A2   | 153   A2   D1.577   IO_L17P_16
B25   | 154   B25   D1.510   IO_L17P_15
AC2   | 155   AC2   D1.442   IO_L17P_14
Y25   | 156   Y25   D1.375   IO_L17P_13
R3   | 157   R3   D1.307   IO_L17P_12
N22   | 158   N22   D1.240   IO_L17P_SM11P_11
AD6   | 159   AD6   D1.712   IO_L17P_18
AC20   | 160   AC20  B1.AB23   VCCO_21
D15   | 161   D15   D1.133   IO_L3P_GC_3
J11   | 162   J11   D1.31   INIT_B_0
J24   | 163   J24   D1.339   IO_L5N_SM4N_13
M13   | 164   M13   D1.12   AVSS_0
T18   | 165   T18   D1.44   R_FUSE_0
G9   | 166   G9   D1.76   IO_L7N_A4_D20_1
V7   | 167   V7   D1.677   IO_L6N_18
G4   | 168   G4   D1.272   IO_L6N_12
H19   | 169   H19   D1.206   IO_L6N_11
A10   | 170   A10   D1.542   IO_L6N_16
AA24   | 171   AA24  D1.611   IO_L6N_17
K1   | 172   K1   D1.407   IO_L6N_14
A19   | 173   A19   D1.476   IO_L6N_15
F17   | 174   F17   D1.146   IO_L9N_GC_3
G14   | 175   G14   D1.61   IO_L0P_A19_1
AA10   | 176   AA10  D1.102   IO_L4P_FCS_B_2
AD3   | 177   AD3   D1.705   IO_L13N_18
W6   | 178   W6   D1.679   IO_L7N_18
J4   | 179   J4   D1.274   IO_L7N_12
J23   | 180   J23   D1.208   IO_L7N_11
Y22   | 181   Y22   D1.613   IO_L7N_17
A8   | 182   A8   D1.544   IO_L7N_16
C18   | 183   C18   D1.478   IO_L7N_15
H2   | 184   H2   D1.409   IO_L7N_14
F25   | 185   F25   D1.329   IO_L0N_SM8N_13
AC22   | 186   AC22  D1.615   IO_L8N_CC_17
Y11   | 187   Y11   D1.95   IO_L0N_CC_RS0_2
AC8   | 188   AC8   D1.166   IO_L3P_GC_D9_4
V12   | 189   V12   D1.57   TMS_0
M25   | 190   M25   D1.344   IO_L8P_CC_SM1P_13
A24   | 191   A24   D1.505   IO_L14N_VREF_15
W1   | 192   W1   D1.437   IO_L14N_VREF_14
U20   | 193   U20   D1.640   IO_L14N_VREF_17
D4   | 194   D4   D1.572   IO_L14N_VREF_16
N19   | 195   N19   D1.235   IO_L14N_VREF_11
U26   | 196   U26   D1.370   IO_L14N_VREF_13
N3   | 197   N3   D1.302   IO_L14N_VREF_12
T24   | 198   T24   D1.367   IO_L13P_13
N7   | 199   N7   D1.299   IO_L13P_12
M22   | 200   M22   D1.232   IO_L13P_11
W21   | 201   W21   D1.637   IO_L13P_17
AB5   | 202   AB5   D1.707   IO_L14N_VREF_18
B22   | 203   B22   D1.502   IO_L13P_15
V2   | 204   V2   D1.434   IO_L13P_14
H18   | 205   H18   D1.78   IO_L8N_CC_A2_D18_1
F24   | 206   F24   D1.328   IO_L0P_SM8P_13
P14   | 207   P14   D1.18   VREFP_0
R23   | 208   R23   D1.243   IO_L18N_SM10N_11
H17   | 209   H17   D1.73   IO_L6P_A7_D23_1
W18   | 210   W18   D1.54   M0_0
AE6   | 211   AE6   D1.716   IO_L19P_18
G11   | 212   G11   D1.72   IO_L5N_A8_D24_1
H24   | 213   H24   D1.338   IO_L5P_SM4P_13
E13   | 214   E13   D1.128   IO_L0N_CC_GC_3
Y10   | 215   Y10   D1.94   IO_L0P_CC_RS1_2
B1   | 216   B1   D1.581   IO_L19P_16
R13   | 217   R13   D1.6   DXN_0
P21   | 218   P21   D1.244   IO_L19P_SM9P_11
B21   | 219   B21   D1.499   IO_L11N_CC_15
K18   | 220   K18   D1.25   VBATT_0
R2   | 221   R2   D1.431   IO_L11N_CC_14
AA12   | 222   AA12  D1.110   IO_L8P_D3_2
A14   | 223   A14   D1.465   IO_L1P_15
F14   | 224   F14   D1.127   IO_L0P_CC_GC_3
AB15   | 225   AB15  D1.104   IO_L5P_FWE_B_2
AD11   | 226   AD11  D1.178   IO_L9P_CC_GC_4
P24   | 227   P24   D1.364   IO_L11N_CC_13
AA17   | 228   AA17  D1.100   IO_L3P_A21_2
R14   | 229   R14   D1.5   DXP_0
AB16   | 230   AB16  D1.105   IO_L5N_CSO_B_2
AC16   | 231   AC16  D1.165   IO_L2N_GC_D10_4
L20   | 232   L20   D1.228   IO_L11P_CC_SM14P_11
H13   | 233   H13   D1.64   IO_L1N_A16_1
D26   | 234   D26   D1.514   IO_L19P_15
AF2   | 235   AF2   D1.446   IO_L19P_14
AA20   | 236   AA20  D1.649   IO_L19P_17
G17   | 237   G17   D1.74   IO_L6N_A6_D22_1
AC26   | 238   AC26  D1.379   IO_L19P_13
P6   | 239   P6   D1.311   IO_L19P_12
N13   | 240   N13   D1.19   VREFN_0
F8   | 241   F8   D1.143   IO_L8P_GC_3
E17   | 242   E17   D1.138   IO_L5N_GC_3
N18   | 243   N18   D1.33   CS_B_0
AC7   | 244   AC7   D1.171   IO_L5N_GC_4
V6   | 245   V6   D1.676   IO_L6P_18
J19   | 246   J19   D1.205   IO_L6P_11
H4   | 247   H4   D1.271   IO_L6P_12
L2   | 248   L2   D1.406   IO_L6P_14
A18   | 249   A18   D1.475   IO_L6P_15
B11   | 250   B11   D1.541   IO_L6P_16
AA23   | 251   AA23  D1.610   IO_L6P_17
P5   | 252   P5   D1.305   IO_L16P_12
W25   | 253   W25   D1.373   IO_L16P_13
C2   | 254   C2   D1.575   IO_L16P_16
Y21   | 255   Y21   D1.643   IO_L16P_17
AB2   | 256   AB2   D1.440   IO_L16P_14
D24   | 257   D24   D1.508   IO_L16P_15
Y3   | 258   Y3   D1.675   IO_L5N_18
AF3   | 259   AF3   D1.710   IO_L16P_18
E15   | 260   E15   D1.134   IO_L3N_GC_3
Y13   | 261   Y13   D1.107   IO_L6N_D6_2
G16   | 262   G16   D1.69   IO_L4P_A11_D27_1
F20   | 263   F20   D1.194   IO_L0N_11
F7   | 264   F7   D1.260   IO_L0N_12
E1   | 265   E1   D1.395   IO_L0N_14
B14   | 266   B14   D1.464   IO_L0N_15
D10   | 267   D10   D1.530   IO_L0N_16
T22   | 268   T22   D1.599   IO_L0N_17
U4   | 269   U4   D1.665   IO_L0N_18
Y6   | 270   Y6   D1.680   IO_L8P_CC_18
K6   | 271   K6   D1.275   IO_L8P_CC_12
AC13   | 272   AC13  D1.176   IO_L8P_CC_GC_4
W10   | 273   W10   D1.60   TDO_0
D8   | 274   D8   D1.545   IO_L8P_CC_16
AC23   | 275   AC23  D1.614   IO_L8P_CC_17
M1   | 276   M1   D1.410   IO_L8P_CC_14
A20   | 277   A20   D1.479   IO_L8P_CC_15
H26   | 278   H26   D1.333   IO_L2N_SM6N_13
E20   | 279   E20   D1.196   IO_L1N_11
E5   | 280   E5   D1.262   IO_L1N_12
A15   | 281   A15   D1.466   IO_L1N_15
E3   | 282   E3   D1.397   IO_L1N_14
R20   | 283   R20   D1.601   IO_L1N_17
C12   | 284   C12   D1.532   IO_L1N_16
T4   | 285   T4   D1.667   IO_L1N_18
V11   | 286   V11   D1.58   TDI_0
N23   | 287   N23   D1.239   IO_L16N_SM12N_11
AA13   | 288   AA13  D1.112   IO_L9P_D1_FS1_2
N24   | 289   N24   D1.347   IO_L9N_CC_SM0N_13
A1   | 290   A1   A1.2   GND
AC11   | 291   AC11  D1.175   IO_L7N_GC_VRP_4
M20   | 292   M20   D1.236   IO_L15P_SM13P_11
E10   | 293   E10   D1.135   IO_L4P_GC_3
AD15   | 294   AD15  D1.168   IO_L4P_GC_4
AA4   | 295   AA4   D1.682   IO_L9P_CC_18
C19   | 296   C19   D1.481   IO_L9P_CC_15
M2   | 297   M2   D1.412   IO_L9P_CC_14
AB24   | 298   AB24  D1.616   IO_L9P_CC_17
B7   | 299   B7   D1.547   IO_L9P_CC_16
K21   | 300   K21   D1.211   IO_L9P_CC_11
N21   | 301   N21   D1.241   IO_L17N_SM11N_11
L7   | 302   L7   D1.277   IO_L9P_CC_12
Y12   | 303   Y12   D1.106   IO_L6P_D7_2
E18   | 304   E18   D1.141   IO_L7P_GC_3
E25   | 305   E25   D1.330   IO_L1P_SM7P_13
R22   | 306   R22   D1.242   IO_L18P_SM10P_11
M24   | 307   M24   D1.346   IO_L9P_CC_SM0P_13
H6   | 308   H6   D1.269   IO_L5P_12
H21   | 309   H21   D1.203   IO_L5P_11
V24   | 310   V24   D1.608   IO_L5P_17
B9   | 311   B9   D1.539   IO_L5P_16
B17   | 312   B17   D1.473   IO_L5P_15
H3   | 313   H3   D1.404   IO_L5P_14
W3   | 314   W3   D1.674   IO_L5P_18
AD10   | 315   AD10  D1.179   IO_L9N_CC_GC_4
K5   | 316   K5   D1.293   IO_L10P_CC_12
P26   | 317   P26   D1.361   IO_L10P_CC_13
P1   | 318   P1   D1.428   IO_L10P_CC_14
D21   | 319   D21   D1.496   IO_L10P_CC_15
D5   | 320   D5   D1.563   IO_L10P_CC_16
AB22   | 321   AB22  D1.631   IO_L10P_CC_17
Y7   | 322   Y7   D1.698   IO_L10P_CC_18
H15   | 323   H15   A1.1   VCCINT
C1   | 324   C1   D1.580   IO_L18N_16
AB19   | 325   AB19  D1.648   IO_L18N_17
AD1   | 326   AD1   D1.445   IO_L18N_14
C26   | 327   C26   D1.513   IO_L18N_15
R5   | 328   R5   D1.310   IO_L18N_12
AA25   | 329   AA25  D1.378   IO_L18N_13
F15   | 330   F15   D1.65   IO_L2P_A15_D31_1
AF4   | 331   AF4   D1.715   IO_L18N_18
T23   | 332   T23   D1.598   IO_L0P_17
L18   | 333   L18   D1.27   HSWAPEN_0
AB11   | 334   AB11  D1.111   IO_L8N_D2_FS2_2
E11   | 335   E11   D1.136   IO_L4N_GC_VREF_3
V23   | 336   V23   D1.609   IO_L5N_17
AD14   | 337   AD14  D1.169   IO_L4N_GC_VREF_4
G1   | 338   G1   D1.398   IO_L2P_14
B15   | 339   B15   D1.467   IO_L2P_15
C13   | 340   C13   D1.533   IO_L2P_16
T20   | 341   T20   D1.602   IO_L2P_17
E22   | 342   E22   D1.197   IO_L2P_11
G6   | 343   G6   D1.263   IO_L2P_12
T7   | 344   T7   D1.668   IO_L2P_18
M19   | 345   M19   D1.237   IO_L15N_SM13N_11
V22   | 346   V22   D1.636   IO_L12N_VRP_17
A5   | 347   A5   D1.568   IO_L12N_VRP_16
C22   | 348   C22   D1.501   IO_L12N_VRP_15
U1   | 349   U1   D1.433   IO_L12N_VRP_14
R26   | 350   R26   D1.366   IO_L12N_VRP_13
M6   | 351   M6   D1.298   IO_L12N_VRP_12
L22   | 352   L22   D1.231   IO_L12N_VRP_11
AC3   | 353   AC3   D1.703   IO_L12N_VRP_18
AB10   | 354   AB10  D1.162   IO_L1P_GC_D13_4
H9   | 355   H9   D1.79   IO_L9P_CC_A1_D17_1
AD5   | 356   AD5   D1.713   IO_L17N_18
A25   | 357   A25   D1.511   IO_L17N_15
AC1   | 358   AC1   D1.443   IO_L17N_14
AC19   | 359   AC19  D1.646   IO_L17N_17
A3   | 360   A3   D1.578   IO_L17N_16
Y26   | 361   Y26   D1.376   IO_L17N_13
T3   | 362   T3   D1.308   IO_L17N_12
C9   | 363   C9   D1.537   IO_L4P_16
Y8   | 364   Y8   D1.98   IO_L2P_A23_2
K3   | 365   K3   D1.402   IO_L4P_14
D18   | 366   D18   D1.471   IO_L4P_15
J6   | 367   J6   D1.267   IO_L4P_12
AA15   | 368   AA15  D1.108   IO_L7P_D5_2
G21   | 369   G21   D1.201   IO_L4P_11
AA9   | 370   AA9   D1.103   IO_L4N_VREF_FOE_B_MOSI_2
V4   | 371   V4   D1.672   IO_L4P_18
AB17   | 372   AB17  D1.101   IO_L3N_A20_2
F22   | 373   F22   D1.199   IO_L3P_11
J1   | 374   J1   D1.408   IO_L7P_14
Y23   | 375   Y23   D1.612   IO_L7P_17
A9   | 376   A9   D1.543   IO_L7P_16
AE3   | 377   AE3   D1.711   IO_L16N_18
F2   | 378   F2   D1.400   IO_L3P_14
U22   | 379   U22   D1.604   IO_L3P_17
A13   | 380   A13   D1.535   IO_L3P_16
AB1   | 381   AB1   D1.441   IO_L16N_14
U5   | 382   U5   D1.670   IO_L3P_18
C3   | 383   C3   D1.576   IO_L16N_16
Y20   | 384   Y20   D1.644   IO_L16N_17
W5   | 385   W5   D1.678   IO_L7P_18
P4   | 386   P4   D1.306   IO_L16N_12
W26   | 387   W26   D1.374   IO_L16N_13
L24   | 388   L24   D1.340   IO_L6P_SM3P_13
E12   | 389   E12   D1.131   IO_L2P_GC_VRN_3
F9   | 390   F9   D1.139   IO_L6P_GC_3
AD13   | 391   AD13  D1.172   IO_L6P_GC_4
D14   | 392   D14   D1.130   IO_L1N_CC_GC_3
G12   | 393   G12   D1.67   IO_L3P_A13_D29_1
H16   | 394   H16   D1.70   IO_L4N_VREF_A10_D26_1
AA5   | 395   AA5   D1.683   IO_L9N_CC_18
AC24   | 396   AC24  D1.617   IO_L9N_CC_17
A7   | 397   A7   D1.548   IO_L9N_CC_16
D19   | 398   D19   D1.482   IO_L9N_CC_15
N2   | 399   N2   D1.413   IO_L9N_CC_14
D13   | 400   D13   D1.129   IO_L1P_CC_GC_3
M7   | 401   M7   D1.278   IO_L9N_CC_12
K20   | 402   K20   D1.212   IO_L9N_CC_11
H12   | 403   H12   D1.68   IO_L3N_A12_D28_1
F13   | 404   F13   D1.62   IO_L0N_A18_1
AB14   | 405   AB14  D1.109   IO_L7N_D4_2
AA3   | 406   AA3   D1.701   IO_L11N_CC_18
T5   | 407   T5   D1.666   IO_L1P_18
R21   | 408   R21   D1.600   IO_L1P_17
C11   | 409   C11   D1.531   IO_L1P_16
AB21   | 410   AB21  D1.634   IO_L11N_CC_17
F3   | 411   F3   D1.396   IO_L1P_14
E6   | 412   E6   D1.261   IO_L1P_12
E21   | 413   E21   D1.195   IO_L1P_11
L3   | 414   L3   D1.296   IO_L11N_CC_12
AB4   | 415   AB4   D1.700   IO_L11P_CC_18
AC21   | 416   AC21  D1.633   IO_L11P_CC_17
C6   | 417   C6   D1.565   IO_L11P_CC_16
C21   | 418   C21   D1.498   IO_L11P_CC_15
T2   | 419   T2   D1.430   IO_L11P_CC_14
P25   | 420   P25   D1.363   IO_L11P_CC_13
L4   | 421   L4   D1.295   IO_L11P_CC_12
M26   | 422   M26   D1.345   IO_L8N_CC_SM1N_13
AA18   | 423   AA18  D1.96   IO_L1P_CC_A25_2
P18   | 424   P18   D1.34   RDWR_B_0
E7   | 425   E7   D1.259   IO_L0P_12
G20   | 426   G20   D1.193   IO_L0P_11
D11   | 427   D11   D1.529   IO_L0P_16
E26   | 428   E26   D1.331   IO_L1N_SM7N_13
E2   | 429   E2   D1.394   IO_L0P_14
C14   | 430   C14   D1.463   IO_L0P_15
A17   | 431   A17   D1.474   IO_L5N_15
J3   | 432   J3   D1.405   IO_L5N_14
V3   | 433   V3   D1.664   IO_L0P_18
B10   | 434   B10   D1.540   IO_L5N_16
H22   | 435   H22   D1.204   IO_L5N_11
G5   | 436   G5   D1.270   IO_L5N_12
J21   | 437   J21   D1.209   IO_L8P_CC_11
N4   | 438   N4   D1.304   IO_L15N_12
H11   | 439   H11   D1.71   IO_L5P_A9_D25_1
G10   | 440   G10   D1.75   IO_L7P_A5_D21_1
E16   | 441   E16   D1.137   IO_L5P_GC_3
AD8   | 442   AD8   D1.170   IO_L5P_GC_4
B5   | 443   B5   D1.569   IO_L13P_16
M14   | 444   M14   D1.11   AVDD_0
[Model Data]
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[End Model Data]
[End Package Model]
|   Model rterm_100
[Model]   rterm_100
Model_type   Series
|   (typ)   (min)   (max)
C_comp   0.0000pF   0.0000pF   0.0000pF
[Temperature Range]   25.0000   85.0000   0.000
[Voltage Range]   2.5000V   2.3750V   2.6250V
[R Series]   103   126   81
| Models and submodels in the file (6): rterm_100 (Series), LVCMOS33_S_12 (I/O), LVCMOS25_F_12 (I/O), LVCMOS25_S_12 (I/O), LVDCI_33 (I/O), LVDS_25 (I/O)
